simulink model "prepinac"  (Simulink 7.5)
settings: Solver=ode45  StartTime=0.0  StopTime=20  FixedStep=1  MaxStep=1  RelTol=1e-3
libraries: commutil2 x32, dspmtrx3 x28, simulink x20
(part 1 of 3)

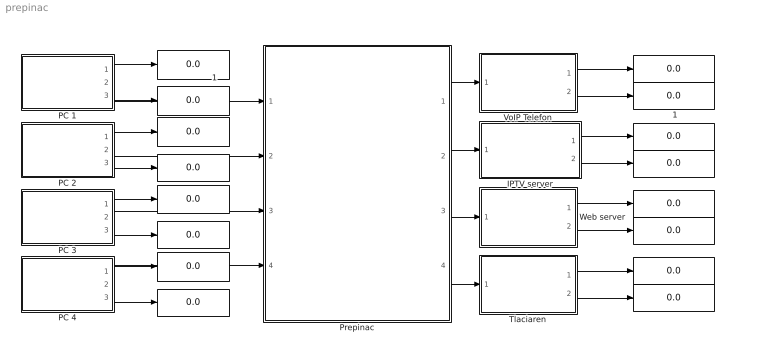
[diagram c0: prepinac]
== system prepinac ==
  " " : Display
  "   " : Display
  "    " : Display
  "     " : Display
  "       " : Display
  "        " : Display
  "          " : Display
  "           " : Display
  "            " : Display
  "                 " : Display
  "                  " : Display
  "                      " : Display
  "                         " : Display
  "                          " : Display
  "                 1" : Display
  " 1" : Display
  IPTV server : Subsystem
  PC 1 : Subsystem
  PC 2 : Subsystem
  PC 3 : Subsystem
  PC 4 : Subsystem
  Prepinac : Subsystem
  Tlaciaren : Subsystem
  VoIP Telefon : Subsystem
  Web server : Subsystem
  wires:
  VoIP Telefon/1(DSCP) -> " "/1
  PC 2/3(MAC) -> "                  "/1
  VoIP Telefon/2(MAC) -> " 1"/1
  IPTV server/2(MAC) -> "     "/1
  Web server/2(MAC) -> "   "/1
  Tlaciaren/2(MAC) -> "        "/1
  IPTV server/1(DSCP) -> "    "/1
  Web server/1(DSCP) -> "          "/1
  Tlaciaren/1(DSCP) -> "            "/1
  PC 1/2(Datovy vystup) -> Prepinac/1(Vstupny port 1)
  PC 4/3(MAC) -> "       "/1
  Prepinac/1(Vystupny port 1) -> VoIP Telefon/1(Vstup)
  Prepinac/3(Vystupny port 3) -> Web server/1(Vstup)
  Prepinac/4(Vystupny port 4) -> Tlaciaren/1(Vstup)
  Prepinac/2(Vystupny port 2) -> IPTV server/1(Vstup)
  PC 3/3(MAC) -> "                         "/1
  PC 1/1(DSCP) -> "                 "/1
  PC 1/3(MAC) -> "                 1"/1
  PC 2/2(Datovy vystup) -> Prepinac/2(Vstupny port 2)
  PC 2/1(DSCP) -> "                      "/1
  PC 3/2(Datovy vystup) -> Prepinac/3(Vstupny port 3)
  PC 3/1(DSCP) -> "                          "/1
  PC 4/1(DSCP) -> "           "/1
  PC 4/2(Datovy vystup) -> Prepinac/4(Vstupny port 4)

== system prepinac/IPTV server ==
  Vstup : Inport  OutDataType=sfix(16)  OutScaling=2^0
  Filtracia DSCP : dspmtrx3/Submatrix  RowSpan=All rows  RowStartMode=Index  RowStartIndex=5  RowEndMode=Index  RowEndIndex=12  ColSpan=Range of columns  ColStartMode=Index  ColStartIndex=113  ColEndMode=Index  ColEndIndex=118
  "MAC adresa " : Constant  Value=[0 0 0 0 0 0 0 0 0 0 1 0 0 1 0 0 1 0 0 1 0 1 1 1 0 0 1 1 0 1 0 0 0 0 0 0 1 1 1 1 1 1 0 0 0 1 0 0]  VectorParams1D=off  OutDataTypeMode=double  OutDataType=sfix(16)  OutScaling=2^0  OutDataTypeStr=double  SampleTime=-1
  Orezanie MAC : dspmtrx3/Submatrix  RowSpan=All rows  RowStartMode=Index  RowStartIndex=5  RowEndMode=Index  RowEndIndex=12  ColSpan=Range of columns  ColStartMode=Index  ColStartIndex=41  ColEndMode=Index  ColEndIndex=48
  Prevod DSCP : commutil2/Bit to Integer Converter  nbits=6  bitOrder=MSB first  signedOutputValues=Unsigned  outDtype=double  outDtypeSigned=Inherit via internal rule
  Prevod MAC : commutil2/Bit to Integer Converter  nbits=8  bitOrder=MSB first  signedOutputValues=Unsigned  outDtype=double  outDtypeSigned=Inherit via internal rule
  DSCP : Outport  OutDataType=sfix(16)  OutScaling=2^0
  MAC : Outport  Port=2  OutDataType=sfix(16)  OutScaling=2^0
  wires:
  Prevod MAC/1 -> MAC/1
  Prevod DSCP/1 -> DSCP/1
  Filtracia DSCP/1 -> Prevod DSCP/1
  Vstup/1 -> Filtracia DSCP/1
  Orezanie MAC/1 -> Prevod MAC/1
  "MAC adresa "/1 -> Orezanie MAC/1

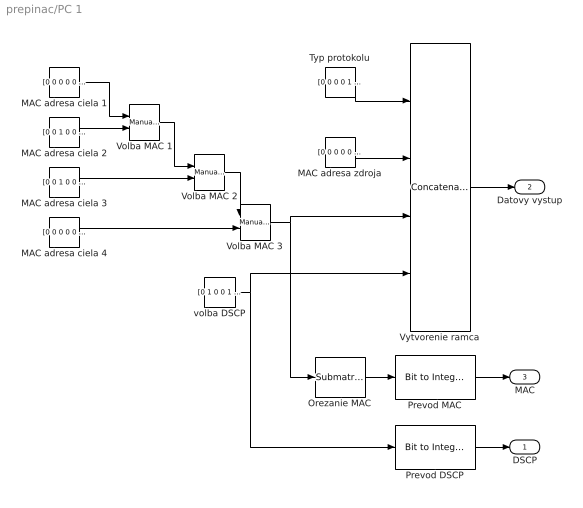
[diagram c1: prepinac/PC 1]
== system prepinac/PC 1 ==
  MAC adresa ciela 1 : Constant  Value=[0 0 0 0 0 0 0 0 0 0 1 0 0 1 0 0 1 0 0 1 0 1 1 1 0 0 1 1 0 1 0 0 0 0 0 0 1 1 1 1 1 1 0 0 0 1 0 0]  VectorParams1D=off  OutDataTypeMode=double  OutDataType=sfix(16)  OutScaling=2^0  OutDataTypeStr=double  SampleTime=-1
  MAC adresa ciela 2 : Constant  Value=[0 0 1 0 0 0 0 0 0 0 0 1 0 1 1 0 1 1 0 1 1 0 0 0 1 1 1 0 0 0 1 1 0 1 1 1 0 0 0 0 1 1 0 0 1 1 1 1]  VectorParams1D=off  OutDataTypeMode=double  OutDataType=sfix(16)  OutScaling=2^0  OutDataTypeStr=double  SampleTime=-1
  MAC adresa ciela 3 : Constant  Value=[0 0 1 0 0 0 0 0 0 0 0 1 0 1 1 0 1 1 0 1 1 0 0 0 1 1 1 0 0 0 1 1 0 1 1 1 0 0 0 0 1 1 0 1 1 1 1 0]  VectorParams1D=off  OutDataTypeMode=double  OutDataType=sfix(16)  OutScaling=2^0  OutDataTypeStr=double  SampleTime=-1
  MAC adresa ciela 4 : Constant  Value=[0 0 0 0 0 0 0 0 0 0 1 1 0 0 0 0 1 1 0 0 0 0 0 1 0 0 1 1 0 0 0 1 0 1 1 1 0 0 1 1 1 0 0 1 1 1 0 1]  VectorParams1D=off  OutDataTypeMode=double  OutDataType=sfix(16)  OutScaling=2^0  OutDataTypeStr=double  SampleTime=-1
  MAC adresa zdroja : Constant  Value=[0 0 0 0 0 0 0 0 0 0 1 0 0 1 0 0 1 0 0 1 0 1 1 1 0 0 1 1 0 1 0 0 0 0 0 0 1 1 1 1 1 1 0 0 0 1 0 1]  VectorParams1D=off  OutDataTypeMode=double  OutDataType=sfix(16)  OutScaling=2^0  OutDataTypeStr=double  SampleTime=-1
  Orezanie MAC : dspmtrx3/Submatrix  RowSpan=All rows  RowStartMode=Index  RowStartIndex=5  RowEndMode=Index  RowEndIndex=12  ColSpan=Range of columns  ColStartMode=Index  ColStartIndex=41  ColEndMode=Index  ColEndIndex=48
  Prevod DSCP : commutil2/Bit to Integer Converter  nbits=6  bitOrder=MSB first  signedOutputValues=Unsigned  outDtype=double  outDtypeSigned=Inherit via internal rule
  Prevod MAC : commutil2/Bit to Integer Converter  nbits=8  bitOrder=MSB first  signedOutputValues=Unsigned  outDtype=double  outDtypeSigned=double
  Typ protokolu : Constant  Value=[0 0 0 0 1 0 0 0 0 0 0 0 0 0 0 0]  VectorParams1D=off  OutDataTypeMode=double  OutDataType=sfix(16)  OutScaling=2^0  OutDataTypeStr=double  SampleTime=-1
  Volba MAC 1 : simulink/Signal Routing/Manual Switch  SystemSampleTime=-1  sw=1  action=0  varsize=off
  Volba MAC 2 : simulink/Signal Routing/Manual Switch  SystemSampleTime=-1  sw=1  action=0  varsize=off
  Volba MAC 3 : simulink/Signal Routing/Manual Switch  SystemSampleTime=-1  sw=1  action=0  varsize=off
  Vytvorenie ramca : Concatenate  NumInputs=4  Mode=Vector
  volba DSCP : Constant  Value=[0 1 0 0 1 0]  VectorParams1D=off  OutDataTypeMode=double  OutDataType=sfix(16)  OutScaling=2^0  OutDataTypeStr=double  SampleTime=-1
  DSCP : Outport  OutDataType=sfix(16)  OutScaling=2^0
  Datovy vystup : Outport  Port=2  OutDataType=sfix(16)  OutScaling=2^0
  MAC : Outport  Port=3  OutDataType=sfix(16)  OutScaling=2^0
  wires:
  Typ protokolu/1 -> Vytvorenie ramca/1
  MAC adresa ciela 2/1 -> Volba MAC 1/2
  MAC adresa ciela 1/1 -> Volba MAC 1/1
  Vytvorenie ramca/1 -> Datovy vystup/1
  MAC adresa ciela 4/1 -> Volba MAC 3/2
  Volba MAC 2/1 -> Volba MAC 3/1
  Volba MAC 1/1 -> Volba MAC 2/1
  MAC adresa ciela 3/1 -> Volba MAC 2/2
  Prevod DSCP/1 -> DSCP/1
  Volba MAC 3/1 -> Vytvorenie ramca/3, Orezanie MAC/1
  Prevod MAC/1 -> MAC/1
  MAC adresa zdroja/1 -> Vytvorenie ramca/2
  volba DSCP/1 -> Vytvorenie ramca/4, Prevod DSCP/1
  Orezanie MAC/1 -> Prevod MAC/1

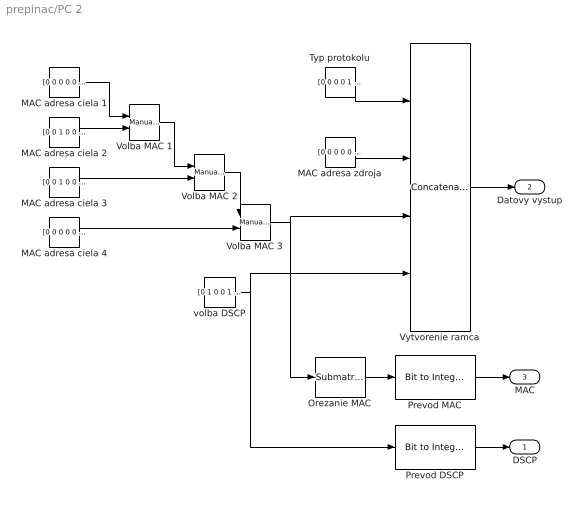
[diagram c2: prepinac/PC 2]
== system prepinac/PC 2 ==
  MAC adresa ciela 1 : Constant  Value=[0 0 0 0 0 0 0 0 0 0 1 0 0 1 0 0 1 0 0 1 0 1 1 1 0 0 1 1 0 1 0 0 0 0 0 0 1 1 1 1 1 1 0 0 0 1 0 0]  VectorParams1D=off  OutDataTypeMode=double  OutDataType=sfix(16)  OutScaling=2^0  OutDataTypeStr=double  SampleTime=-1
  MAC adresa ciela 2 : Constant  Value=[0 0 1 0 0 0 0 0 0 0 0 1 0 1 1 0 1 1 0 1 1 0 0 0 1 1 1 0 0 0 1 1 0 1 1 1 0 0 0 0 1 1 0 0 1 1 1 1]  VectorParams1D=off  OutDataTypeMode=double  OutDataType=sfix(16)  OutScaling=2^0  OutDataTypeStr=double  SampleTime=-1
  MAC adresa ciela 3 : Constant  Value=[0 0 1 0 0 0 0 0 0 0 0 1 0 1 1 0 1 1 0 1 1 0 0 0 1 1 1 0 0 0 1 1 0 1 1 1 0 0 0 0 1 1 0 1 1 1 1 0]  VectorParams1D=off  OutDataTypeMode=double  OutDataType=sfix(16)  OutScaling=2^0  OutDataTypeStr=double  SampleTime=-1
  MAC adresa ciela 4 : Constant  Value=[0 0 0 0 0 0 0 0 0 0 1 1 0 0 0 0 1 1 0 0 0 0 0 1 0 0 1 1 0 0 0 1 0 1 1 1 0 0 1 1 1 0 0 1 1 1 0 1]  VectorParams1D=off  OutDataTypeMode=double  OutDataType=sfix(16)  OutScaling=2^0  OutDataTypeStr=double  SampleTime=-1
  MAC adresa zdroja : Constant  Value=[0 0 0 0 0 0 0 0 0 0 1 0 0 1 0 0 1 0 0 1 0 1 1 1 0 0 1 1 0 1 0 0 0 0 0 0 1 1 1 1 1 1 0 0 0 1 0 1]  VectorParams1D=off  OutDataTypeMode=double  OutDataType=sfix(16)  OutScaling=2^0  OutDataTypeStr=double  SampleTime=-1
  Orezanie MAC : dspmtrx3/Submatrix  RowSpan=All rows  RowStartMode=Index  RowStartIndex=5  RowEndMode=Index  RowEndIndex=12  ColSpan=Range of columns  ColStartMode=Index  ColStartIndex=41  ColEndMode=Index  ColEndIndex=48
  Prevod DSCP : commutil2/Bit to Integer Converter  nbits=6  bitOrder=MSB first  signedOutputValues=Unsigned  outDtype=double  outDtypeSigned=Inherit via internal rule
  Prevod MAC : commutil2/Bit to Integer Converter  nbits=8  bitOrder=MSB first  signedOutputValues=Unsigned  outDtype=double  outDtypeSigned=double
  Typ protokolu : Constant  Value=[0 0 0 0 1 0 0 0 0 0 0 0 0 0 0 0]  VectorParams1D=off  OutDataTypeMode=double  OutDataType=sfix(16)  OutScaling=2^0  OutDataTypeStr=double  SampleTime=-1
  Volba MAC 1 : simulink/Signal Routing/Manual Switch  SystemSampleTime=-1  sw=1  action=0  varsize=off
  Volba MAC 2 : simulink/Signal Routing/Manual Switch  SystemSampleTime=-1  sw=1  action=0  varsize=off
  Volba MAC 3 : simulink/Signal Routing/Manual Switch  SystemSampleTime=-1  sw=1  action=0  varsize=off
  Vytvorenie ramca : Concatenate  NumInputs=4  Mode=Vector
  volba DSCP : Constant  Value=[0 1 0 0 1 0]  VectorParams1D=off  OutDataTypeMode=double  OutDataType=sfix(16)  OutScaling=2^0  OutDataTypeStr=double  SampleTime=-1
  DSCP : Outport  OutDataType=sfix(16)  OutScaling=2^0
  Datovy vystup : Outport  Port=2  OutDataType=sfix(16)  OutScaling=2^0
  MAC : Outport  Port=3  OutDataType=sfix(16)  OutScaling=2^0
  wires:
  Orezanie MAC/1 -> Prevod MAC/1
  volba DSCP/1 -> Prevod DSCP/1, Vytvorenie ramca/4
  MAC adresa zdroja/1 -> Vytvorenie ramca/2
  Prevod MAC/1 -> MAC/1
  Volba MAC 3/1 -> Orezanie MAC/1, Vytvorenie ramca/3
  Prevod DSCP/1 -> DSCP/1
  MAC adresa ciela 3/1 -> Volba MAC 2/2
  Volba MAC 1/1 -> Volba MAC 2/1
  Volba MAC 2/1 -> Volba MAC 3/1
  MAC adresa ciela 4/1 -> Volba MAC 3/2
  Vytvorenie ramca/1 -> Datovy vystup/1
  MAC adresa ciela 1/1 -> Volba MAC 1/1
  MAC adresa ciela 2/1 -> Volba MAC 1/2
  Typ protokolu/1 -> Vytvorenie ramca/1

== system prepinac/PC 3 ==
  MAC adresa ciela 1 : Constant  Value=[0 0 0 0 0 0 0 0 0 0 1 0 0 1 0 0 1 0 0 1 0 1 1 1 0 0 1 1 0 1 0 0 0 0 0 0 1 1 1 1 1 1 0 0 0 1 0 0]  VectorParams1D=off  OutDataTypeMode=double  OutDataType=sfix(16)  OutScaling=2^0  OutDataTypeStr=double  SampleTime=-1
  MAC adresa ciela 2 : Constant  Value=[0 0 1 0 0 0 0 0 0 0 0 1 0 1 1 0 1 1 0 1 1 0 0 0 1 1 1 0 0 0 1 1 0 1 1 1 0 0 0 0 1 1 0 0 1 1 1 1]  VectorParams1D=off  OutDataTypeMode=double  OutDataType=sfix(16)  OutScaling=2^0  OutDataTypeStr=double  SampleTime=-1
  MAC adresa ciela 3 : Constant  Value=[0 0 1 0 0 0 0 0 0 0 0 1 0 1 1 0 1 1 0 1 1 0 0 0 1 1 1 0 0 0 1 1 0 1 1 1 0 0 0 0 1 1 0 1 1 1 1 0]  VectorParams1D=off  OutDataTypeMode=double  OutDataType=sfix(16)  OutScaling=2^0  OutDataTypeStr=double  SampleTime=-1
  MAC adresa ciela 4 : Constant  Value=[0 0 0 0 0 0 0 0 0 0 1 1 0 0 0 0 1 1 0 0 0 0 0 1 0 0 1 1 0 0 0 1 0 1 1 1 0 0 1 1 1 0 0 1 1 1 0 1]  VectorParams1D=off  OutDataTypeMode=double  OutDataType=sfix(16)  OutScaling=2^0  OutDataTypeStr=double  SampleTime=-1
  MAC adresa zdroja : Constant  Value=[0 0 0 0 0 0 0 0 0 0 1 0 0 1 0 0 1 0 0 1 0 1 1 1 0 0 1 1 0 1 0 0 0 0 0 0 1 1 1 1 1 1 0 0 0 1 0 1]  VectorParams1D=off  OutDataTypeMode=double  OutDataType=sfix(16)  OutScaling=2^0  OutDataTypeStr=double  SampleTime=-1
  Orezanie MAC : dspmtrx3/Submatrix  RowSpan=All rows  RowStartMode=Index  RowStartIndex=5  RowEndMode=Index  RowEndIndex=12  ColSpan=Range of columns  ColStartMode=Index  ColStartIndex=41  ColEndMode=Index  ColEndIndex=48
  Prevod DSCP : commutil2/Bit to Integer Converter  nbits=6  bitOrder=MSB first  signedOutputValues=Unsigned  outDtype=double  outDtypeSigned=Inherit via internal rule
  Prevod MAC : commutil2/Bit to Integer Converter  nbits=8  bitOrder=MSB first  signedOutputValues=Unsigned  outDtype=double  outDtypeSigned=double
  Typ protokolu : Constant  Value=[0 0 0 0 1 0 0 0 0 0 0 0 0 0 0 0]  VectorParams1D=off  OutDataTypeMode=double  OutDataType=sfix(16)  OutScaling=2^0  OutDataTypeStr=double  SampleTime=-1
  Volba MAC 1 : simulink/Signal Routing/Manual Switch  SystemSampleTime=-1  sw=1  action=0  varsize=off
  Volba MAC 2 : simulink/Signal Routing/Manual Switch  SystemSampleTime=-1  sw=1  action=0  varsize=off
  Volba MAC 3 : simulink/Signal Routing/Manual Switch  SystemSampleTime=-1  sw=1  action=0  varsize=off
  Vytvorenie ramca : Concatenate  NumInputs=4  Mode=Vector
  volba DSCP : Constant  Value=[0 1 0 0 1 0]  VectorParams1D=off  OutDataTypeMode=double  OutDataType=sfix(16)  OutScaling=2^0  OutDataTypeStr=double  SampleTime=-1
  DSCP : Outport  OutDataType=sfix(16)  OutScaling=2^0
  Datovy vystup : Outport  Port=2  OutDataType=sfix(16)  OutScaling=2^0
  MAC : Outport  Port=3  OutDataType=sfix(16)  OutScaling=2^0
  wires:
  Typ protokolu/1 -> Vytvorenie ramca/1
  MAC adresa ciela 2/1 -> Volba MAC 1/2
  MAC adresa ciela 1/1 -> Volba MAC 1/1
  Vytvorenie ramca/1 -> Datovy vystup/1
  MAC adresa ciela 4/1 -> Volba MAC 3/2
  Volba MAC 2/1 -> Volba MAC 3/1
  Volba MAC 1/1 -> Volba MAC 2/1
  MAC adresa ciela 3/1 -> Volba MAC 2/2
  Prevod DSCP/1 -> DSCP/1
  Volba MAC 3/1 -> Vytvorenie ramca/3, Orezanie MAC/1
  Prevod MAC/1 -> MAC/1
  MAC adresa zdroja/1 -> Vytvorenie ramca/2
  volba DSCP/1 -> Vytvorenie ramca/4, Prevod DSCP/1
  Orezanie MAC/1 -> Prevod MAC/1

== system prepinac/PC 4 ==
  MAC adresa ciela 1 : Constant  Value=[0 0 0 0 0 0 0 0 0 0 1 0 0 1 0 0 1 0 0 1 0 1 1 1 0 0 1 1 0 1 0 0 0 0 0 0 1 1 1 1 1 1 0 0 0 1 0 0]  VectorParams1D=off  OutDataTypeMode=double  OutDataType=sfix(16)  OutScaling=2^0  OutDataTypeStr=double  SampleTime=-1
  MAC adresa ciela 2 : Constant  Value=[0 0 1 0 0 0 0 0 0 0 0 1 0 1 1 0 1 1 0 1 1 0 0 0 1 1 1 0 0 0 1 1 0 1 1 1 0 0 0 0 1 1 0 0 1 1 1 1]  VectorParams1D=off  OutDataTypeMode=double  OutDataType=sfix(16)  OutScaling=2^0  OutDataTypeStr=double  SampleTime=-1
  MAC adresa ciela 3 : Constant  Value=[0 0 1 0 0 0 0 0 0 0 0 1 0 1 1 0 1 1 0 1 1 0 0 0 1 1 1 0 0 0 1 1 0 1 1 1 0 0 0 0 1 1 0 1 1 1 1 0]  VectorParams1D=off  OutDataTypeMode=double  OutDataType=sfix(16)  OutScaling=2^0  OutDataTypeStr=double  SampleTime=-1
  MAC adresa ciela 4 : Constant  Value=[0 0 0 0 0 0 0 0 0 0 1 1 0 0 0 0 1 1 0 0 0 0 0 1 0 0 1 1 0 0 0 1 0 1 1 1 0 0 1 1 1 0 0 1 1 1 0 1]  VectorParams1D=off  OutDataTypeMode=double  OutDataType=sfix(16)  OutScaling=2^0  OutDataTypeStr=double  SampleTime=-1
  MAC adresa zdroja : Constant  Value=[0 0 0 0 0 0 0 0 0 0 1 0 0 1 0 0 1 0 0 1 0 1 1 1 0 0 1 1 0 1 0 0 0 0 0 0 1 1 1 1 1 1 0 0 0 1 0 1]  VectorParams1D=off  OutDataTypeMode=double  OutDataType=sfix(16)  OutScaling=2^0  OutDataTypeStr=double  SampleTime=-1
  Orezanie MAC : dspmtrx3/Submatrix  RowSpan=All rows  RowStartMode=Index  RowStartIndex=5  RowEndMode=Index  RowEndIndex=12  ColSpan=Range of columns  ColStartMode=Index  ColStartIndex=41  ColEndMode=Index  ColEndIndex=48
  Prevod DSCP : commutil2/Bit to Integer Converter  nbits=6  bitOrder=MSB first  signedOutputValues=Unsigned  outDtype=double  outDtypeSigned=Inherit via internal rule
  Prevod MAC : commutil2/Bit to Integer Converter  nbits=8  bitOrder=MSB first  signedOutputValues=Unsigned  outDtype=double  outDtypeSigned=double
  Typ protokolu : Constant  Value=[0 0 0 0 1 0 0 0 0 0 0 0 0 0 0 0]  VectorParams1D=off  OutDataTypeMode=double  OutDataType=sfix(16)  OutScaling=2^0  OutDataTypeStr=double  SampleTime=-1
  Volba MAC 1 : simulink/Signal Routing/Manual Switch  SystemSampleTime=-1  sw=1  action=0  varsize=off
  Volba MAC 2 : simulink/Signal Routing/Manual Switch  SystemSampleTime=-1  sw=1  action=0  varsize=off
  Volba MAC 3 : simulink/Signal Routing/Manual Switch  SystemSampleTime=-1  sw=1  action=0  varsize=off
  Vytvorenie ramca : Concatenate  NumInputs=4  Mode=Vector
  volba DSCP : Constant  Value=[0 1 0 0 1 0]  VectorParams1D=off  OutDataTypeMode=double  OutDataType=sfix(16)  OutScaling=2^0  OutDataTypeStr=double  SampleTime=-1
  DSCP : Outport  OutDataType=sfix(16)  OutScaling=2^0
  Datovy vystup : Outport  Port=2  OutDataType=sfix(16)  OutScaling=2^0
  MAC : Outport  Port=3  OutDataType=sfix(16)  OutScaling=2^0
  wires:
  Orezanie MAC/1 -> Prevod MAC/1
  volba DSCP/1 -> Prevod DSCP/1, Vytvorenie ramca/4
  MAC adresa zdroja/1 -> Vytvorenie ramca/2
  Prevod MAC/1 -> MAC/1
  Volba MAC 3/1 -> Orezanie MAC/1, Vytvorenie ramca/3
  Prevod DSCP/1 -> DSCP/1
  MAC adresa ciela 3/1 -> Volba MAC 2/2
  Volba MAC 1/1 -> Volba MAC 2/1
  Volba MAC 2/1 -> Volba MAC 3/1
  MAC adresa ciela 4/1 -> Volba MAC 3/2
  Vytvorenie ramca/1 -> Datovy vystup/1
  MAC adresa ciela 1/1 -> Volba MAC 1/1
  MAC adresa ciela 2/1 -> Volba MAC 1/2
  Typ protokolu/1 -> Vytvorenie ramca/1

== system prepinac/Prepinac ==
  Vstupny port 1 : Inport  OutDataType=sfix(16)  OutScaling=2^0
  Vstupny port 2 : Inport  Port=2  OutDataType=sfix(16)  OutScaling=2^0
  Vstupny port 3 : Inport  Port=3  OutDataType=sfix(16)  OutScaling=2^0
  Vstupny port 4 : Inport  Port=4  OutDataType=sfix(16)  OutScaling=2^0
  Riadenie QoS : Subsystem
  Riadenie prepinania : Subsystem
  Vystupny port 1 : Outport  OutDataType=sfix(16)  OutScaling=2^0
  Vystupny port 2 : Outport  Port=2  OutDataType=sfix(16)  OutScaling=2^0
  Vystupny port 3 : Outport  Port=3  OutDataType=sfix(16)  OutScaling=2^0
  Vystupny port 4 : Outport  Port=4  OutDataType=sfix(16)  OutScaling=2^0
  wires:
  Vstupny port 1/1 -> Riadenie QoS/1(In1), Riadenie prepinania/1(MAC1)
  Vstupny port 2/1 -> Riadenie QoS/2(In2), Riadenie prepinania/2(MAC2)
  Vstupny port 3/1 -> Riadenie QoS/3(In3), Riadenie prepinania/3(MAC3)
  Vstupny port 4/1 -> Riadenie QoS/4(In4), Riadenie prepinania/4(MAC4)
  Riadenie QoS/1(Datovy vystup) -> Riadenie prepinania/5(Data)
  Riadenie prepinania/4(Vystup4) -> Vystupny port 4/1
  Riadenie prepinania/3(Vystup3) -> Vystupny port 3/1
  Riadenie prepinania/2(Vystup2) -> Vystupny port 2/1
  Riadenie prepinania/1(Vystup1) -> Vystupny port 1/1

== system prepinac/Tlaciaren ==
  Vstup : Inport  OutDataType=sfix(16)  OutScaling=2^0
  Filtracia DSCP : dspmtrx3/Submatrix  RowSpan=All rows  RowStartMode=Index  RowStartIndex=5  RowEndMode=Index  RowEndIndex=12  ColSpan=Range of columns  ColStartMode=Index  ColStartIndex=113  ColEndMode=Index  ColEndIndex=118
  "MAC adresa " : Constant  Value=[0 0 0 0 0 0 0 0 0 0 1 0 0 1 0 0 1 0 0 1 0 1 1 1 0 0 1 1 0 1 0 0 0 0 0 0 1 1 1 1 1 1 0 0 0 1 0 0]  VectorParams1D=off  OutDataTypeMode=double  OutDataType=sfix(16)  OutScaling=2^0  OutDataTypeStr=double  SampleTime=-1
  Orezanie MAC : dspmtrx3/Submatrix  RowSpan=All rows  RowStartMode=Index  RowStartIndex=5  RowEndMode=Index  RowEndIndex=12  ColSpan=Range of columns  ColStartMode=Index  ColStartIndex=41  ColEndMode=Index  ColEndIndex=48
  Prevod DSCP : commutil2/Bit to Integer Converter  nbits=6  bitOrder=MSB first  signedOutputValues=Unsigned  outDtype=double  outDtypeSigned=Inherit via internal rule
  Prevod MAC : commutil2/Bit to Integer Converter  nbits=8  bitOrder=MSB first  signedOutputValues=Unsigned  outDtype=double  outDtypeSigned=Inherit via internal rule
  DSCP : Outport  OutDataType=sfix(16)  OutScaling=2^0
  MAC : Outport  Port=2  OutDataType=sfix(16)  OutScaling=2^0
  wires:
  Prevod MAC/1 -> MAC/1
  Prevod DSCP/1 -> DSCP/1
  Filtracia DSCP/1 -> Prevod DSCP/1
  Vstup/1 -> Filtracia DSCP/1
  Orezanie MAC/1 -> Prevod MAC/1
  "MAC adresa "/1 -> Orezanie MAC/1

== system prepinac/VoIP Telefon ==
  Vstup : Inport  OutDataType=sfix(16)  OutScaling=2^0
  Filtracia DSCP : dspmtrx3/Submatrix  RowSpan=All rows  RowStartMode=Index  RowStartIndex=5  RowEndMode=Index  RowEndIndex=12  ColSpan=Range of columns  ColStartMode=Index  ColStartIndex=113  ColEndMode=Index  ColEndIndex=118
  "MAC adresa " : Constant  Value=[0 0 0 0 0 0 0 0 0 0 1 0 0 1 0 0 1 0 0 1 0 1 1 1 0 0 1 1 0 1 0 0 0 0 0 0 1 1 1 1 1 1 0 0 0 1 0 0]  VectorParams1D=off  OutDataTypeMode=double  OutDataType=sfix(16)  OutScaling=2^0  OutDataTypeStr=double  SampleTime=-1
  Orezanie MAC : dspmtrx3/Submatrix  RowSpan=All rows  RowStartMode=Index  RowStartIndex=5  RowEndMode=Index  RowEndIndex=12  ColSpan=Range of columns  ColStartMode=Index  ColStartIndex=41  ColEndMode=Index  ColEndIndex=48
  Prevod DSCP : commutil2/Bit to Integer Converter  nbits=6  bitOrder=MSB first  signedOutputValues=Unsigned  outDtype=double  outDtypeSigned=Inherit via internal rule
  Prevod MAC : commutil2/Bit to Integer Converter  nbits=8  bitOrder=MSB first  signedOutputValues=Unsigned  outDtype=double  outDtypeSigned=Inherit via internal rule
  DSCP : Outport  OutDataType=sfix(16)  OutScaling=2^0
  MAC : Outport  Port=2  OutDataType=sfix(16)  OutScaling=2^0
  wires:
  "MAC adresa "/1 -> Orezanie MAC/1
  Orezanie MAC/1 -> Prevod MAC/1
  Vstup/1 -> Filtracia DSCP/1
  Filtracia DSCP/1 -> Prevod DSCP/1
  Prevod DSCP/1 -> DSCP/1
  Prevod MAC/1 -> MAC/1

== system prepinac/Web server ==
  Vstup : Inport  OutDataType=sfix(16)  OutScaling=2^0
  Filtracia DSCP : dspmtrx3/Submatrix  RowSpan=All rows  RowStartMode=Index  RowStartIndex=5  RowEndMode=Index  RowEndIndex=12  ColSpan=Range of columns  ColStartMode=Index  ColStartIndex=113  ColEndMode=Index  ColEndIndex=118
  "MAC adresa " : Constant  Value=[0 0 0 0 0 0 0 0 0 0 1 0 0 1 0 0 1 0 0 1 0 1 1 1 0 0 1 1 0 1 0 0 0 0 0 0 1 1 1 1 1 1 0 0 0 1 0 0]  VectorParams1D=off  OutDataTypeMode=double  OutDataType=sfix(16)  OutScaling=2^0  OutDataTypeStr=double  SampleTime=-1
  Orezanie MAC : dspmtrx3/Submatrix  RowSpan=All rows  RowStartMode=Index  RowStartIndex=5  RowEndMode=Index  RowEndIndex=12  ColSpan=Range of columns  ColStartMode=Index  ColStartIndex=41  ColEndMode=Index  ColEndIndex=48
  Prevod DSCP : commutil2/Bit to Integer Converter  nbits=6  bitOrder=MSB first  signedOutputValues=Unsigned  outDtype=double  outDtypeSigned=Inherit via internal rule
  Prevod MAC : commutil2/Bit to Integer Converter  nbits=8  bitOrder=MSB first  signedOutputValues=Unsigned  outDtype=double  outDtypeSigned=Inherit via internal rule
  DSCP : Outport  OutDataType=sfix(16)  OutScaling=2^0
  MAC : Outport  Port=2  OutDataType=sfix(16)  OutScaling=2^0
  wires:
  "MAC adresa "/1 -> Orezanie MAC/1
  Orezanie MAC/1 -> Prevod MAC/1
  Vstup/1 -> Filtracia DSCP/1
  Filtracia DSCP/1 -> Prevod DSCP/1
  Prevod DSCP/1 -> DSCP/1
  Prevod MAC/1 -> MAC/1

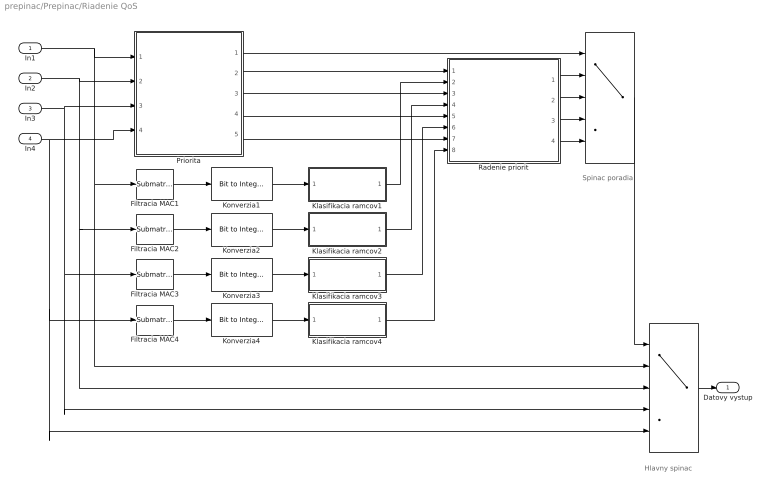
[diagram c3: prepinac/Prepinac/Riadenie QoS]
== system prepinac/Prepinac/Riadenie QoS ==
  note: Hlavny spinac
  note: Spinac poradia
  In1 : Inport  OutDataType=sfix(16)  OutScaling=2^0
  In2 : Inport  Port=2  OutDataType=sfix(16)  OutScaling=2^0
  In3 : Inport  Port=3  OutDataType=sfix(16)  OutScaling=2^0
  In4 : Inport  Port=4  OutDataType=sfix(16)  OutScaling=2^0
  "   " : MultiPortSwitch  DataPortOrder=Zero-based contiguous  Inputs=4  zeroidx=on
  "         " : MultiPortSwitch  Inputs=4  zeroidx=off
  Filtracia MAC{1..4} (4 alike) : dspmtrx3/Submatrix  RowSpan=All rows  RowStartMode=Index  RowStartIndex=5  RowEndMode=Index  RowEndIndex=12  ColSpan=Range of columns  ColStartMode=Index  ColStartIndex=105  ColEndMode=Index  ColEndIndex=112
  Klasifikacia ramcov1 : Subsystem
  Klasifikacia ramcov2 : Subsystem
  Klasifikacia ramcov3 : Subsystem
  Klasifikacia ramcov4 : Subsystem
  Konverzia{1..4} (4 alike) : commutil2/Bit to Integer Converter  nbits=8  bitOrder=MSB first  signedOutputValues=Unsigned  outDtype=Same as input  outDtypeSigned=Inherit via internal rule
  Priorita : Subsystem
  Radenie priorit : Subsystem
  Datovy vystup : Outport  OutDataType=sfix(16)  OutScaling=2^0
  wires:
  In1/1 -> Priorita/1(In1), "         "/2, Filtracia MAC1/1
  In2/1 -> Priorita/2(In2), "         "/3, Filtracia MAC2/1
  In3/1 -> Priorita/3(In3), "         "/4, Filtracia MAC3/1
  In4/1 -> Priorita/4(In4), "         "/5, Filtracia MAC4/1
  "         "/1 -> Datovy vystup/1
  Priorita/2(Out1) -> Radenie priorit/1(vst1)
  Priorita/3(Out2) -> Radenie priorit/3(vst2)
  Priorita/4(Out3) -> Radenie priorit/5(vst3)
  Priorita/5(Out4) -> Radenie priorit/7(vst4)
  Priorita/1(Trg1) -> "   "/1
  Radenie priorit/1(sig1) -> "   "/2
  Radenie priorit/2(sig2) -> "   "/3
  Radenie priorit/3(sig3) -> "   "/4
  Radenie priorit/4(sig4) -> "   "/5
  "   "/1 -> "         "/1
  Filtracia MAC1/1 -> Konverzia1/1
  Filtracia MAC2/1 -> Konverzia2/1
  Filtracia MAC3/1 -> Konverzia3/1
  Filtracia MAC4/1 -> Konverzia4/1
  Konverzia1/1 -> Klasifikacia ramcov1/1(In)
  Konverzia2/1 -> Klasifikacia ramcov2/1(In)
  Konverzia3/1 -> Klasifikacia ramcov3/1(In)
  Konverzia4/1 -> Klasifikacia ramcov4/1(In)
  Klasifikacia ramcov4/1(Out) -> Radenie priorit/8(adr4)
  Klasifikacia ramcov3/1(Out) -> Radenie priorit/6(adr3)
  Klasifikacia ramcov2/1(Out) -> Radenie priorit/4(adr2)
  Klasifikacia ramcov1/1(Out) -> Radenie priorit/2(adr1)

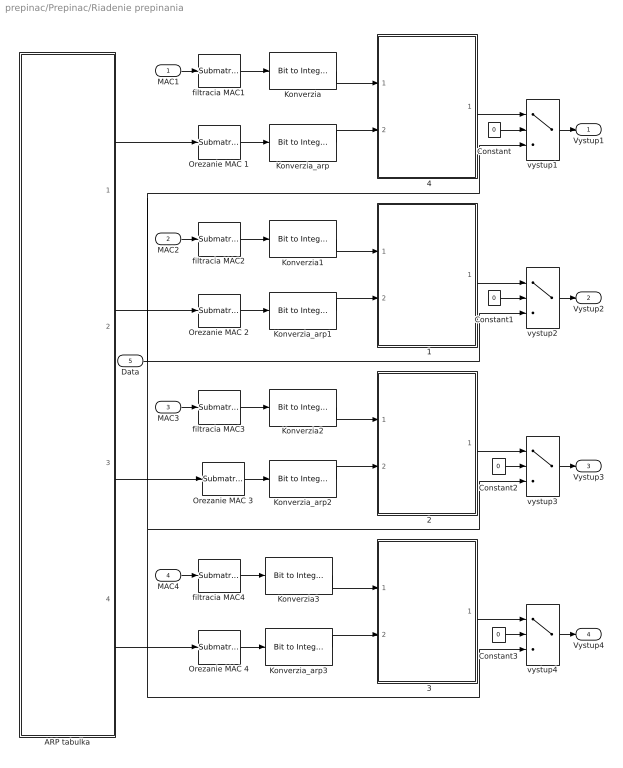
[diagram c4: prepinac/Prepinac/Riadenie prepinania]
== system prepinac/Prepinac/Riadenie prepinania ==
  MAC1 : Inport  OutDataType=sfix(16)  OutScaling=2^0
  MAC2 : Inport  Port=2  OutDataType=sfix(16)  OutScaling=2^0
  MAC3 : Inport  Port=3  OutDataType=sfix(16)  OutScaling=2^0
  MAC4 : Inport  Port=4  OutDataType=sfix(16)  OutScaling=2^0
  Data : Inport  Port=5  OutDataType=sfix(16)  OutScaling=2^0
  "  1" : Stateflow chart  TreatAsAtomicUnit=on
  "  2" : Stateflow chart  TreatAsAtomicUnit=on
  "  3" : Stateflow chart  TreatAsAtomicUnit=on
  "  4" : Stateflow chart  TreatAsAtomicUnit=on
  ARP tabulka : Subsystem
  Constant{,1..3} (4 alike) : Constant  Value=0  OutDataType=sfix(16)  OutScaling=2^0
  Konverzia{,1..3} (4 alike) : commutil2/Bit to Integer Converter  nbits=8  bitOrder=MSB first  signedOutputValues=Unsigned  outDtype=Same as input  outDtypeSigned=Inherit via internal rule
  Konverzia_arp{,1..3} (4 alike) : commutil2/Bit to Integer Converter  nbits=8  bitOrder=MSB first  signedOutputValues=Unsigned  outDtype=double  outDtypeSigned=Inherit via internal rule
  Orezanie MAC {1..4} (4 alike) : dspmtrx3/Submatrix  RowSpan=All rows  RowStartMode=Index  RowStartIndex=5  RowEndMode=Index  RowEndIndex=12  ColSpan=Range of columns  ColStartMode=Index  ColStartIndex=41  ColEndMode=Index  ColEndIndex=48
  filtracia MAC{1..4} (4 alike) : dspmtrx3/Submatrix  RowSpan=All rows  RowStartMode=Index  RowStartIndex=5  RowEndMode=Index  RowEndIndex=12  ColSpan=Range of columns  ColStartMode=Index  ColStartIndex=105  ColEndMode=Index  ColEndIndex=112
  vystup{1..4} (4 alike) : MultiPortSwitch  Inputs=2  zeroidx=off
  Vystup1 : Outport  OutDataType=sfix(16)  OutScaling=2^0
  Vystup2 : Outport  Port=2  OutDataType=sfix(16)  OutScaling=2^0
  Vystup3 : Outport  Port=3  OutDataType=sfix(16)  OutScaling=2^0
  Vystup4 : Outport  Port=4  OutDataType=sfix(16)  OutScaling=2^0
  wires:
  vystup2/1 -> Vystup2/1
  vystup1/1 -> Vystup1/1
  Data/1 -> vystup1/3, vystup3/3, vystup4/3, vystup2/3
  vystup3/1 -> Vystup3/1
  vystup4/1 -> Vystup4/1
  Constant/1 -> vystup1/2
  Constant1/1 -> vystup2/2
  Orezanie MAC 1/1 -> Konverzia_arp/1
  Orezanie MAC 2/1 -> Konverzia_arp1/1
  Orezanie MAC 3/1 -> Konverzia_arp2/1
  Orezanie MAC 4/1 -> Konverzia_arp3/1
  ARP tabulka/1(MAC adresa 1) -> Orezanie MAC 1/1
  ARP tabulka/4(MAC adresa 4) -> Orezanie MAC 4/1
  ARP tabulka/3(MAC adresa 3) -> Orezanie MAC 3/1
  ARP tabulka/2(MAC adresa 2) -> Orezanie MAC 2/1
  filtracia MAC1/1 -> Konverzia/1
  filtracia MAC2/1 -> Konverzia1/1
  filtracia MAC3/1 -> Konverzia2/1
  filtracia MAC4/1 -> Konverzia3/1
  Konverzia1/1 -> "  1"/1(MAC_prijata)
  Konverzia2/1 -> "  2"/1(MAC_prijata)
  Konverzia3/1 -> "  3"/1(MAC_prijata)
  MAC1/1 -> filtracia MAC1/1
  MAC2/1 -> filtracia MAC2/1
  MAC3/1 -> filtracia MAC3/1
  MAC4/1 -> filtracia MAC4/1
  Konverzia_arp2/1 -> "  2"/2(MAC_arp)
  Konverzia_arp1/1 -> "  1"/2(MAC_arp)
  Konverzia_arp/1 -> "  4"/2(MAC_arp)
  Konverzia/1 -> "  4"/1(MAC_prijata)
  "  4"/1(y) -> vystup1/1
  Konverzia_arp3/1 -> "  3"/2(MAC_arp)
  "  1"/1(y) -> vystup2/1
  "  2"/1(y) -> vystup3/1
  Constant2/1 -> vystup3/2
  "  3"/1(y) -> vystup4/1
  Constant3/1 -> vystup4/2

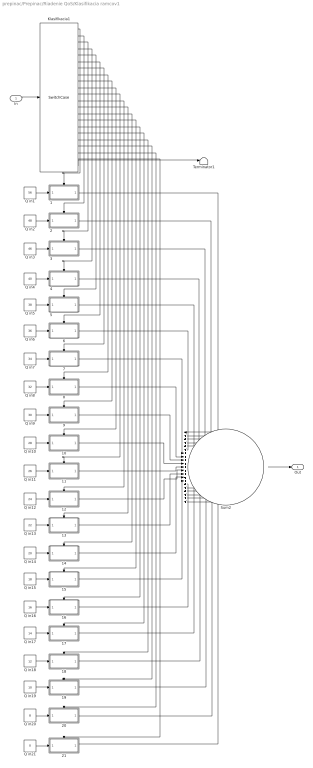
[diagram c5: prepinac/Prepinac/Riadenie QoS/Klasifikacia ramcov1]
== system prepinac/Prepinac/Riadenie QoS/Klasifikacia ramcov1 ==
  In : Inport  OutDataType=sfix(16)  OutScaling=2^0
  1 : Subsystem  TreatAsAtomicUnit=on
  10 : Subsystem  TreatAsAtomicUnit=on
  11 : Subsystem  TreatAsAtomicUnit=on
  12 : Subsystem  TreatAsAtomicUnit=on
  13 : Subsystem  TreatAsAtomicUnit=on
  14 : Subsystem  TreatAsAtomicUnit=on
  15 : Subsystem  TreatAsAtomicUnit=on
  16 : Subsystem  TreatAsAtomicUnit=on
  17 : Subsystem  TreatAsAtomicUnit=on
  18 : Subsystem  TreatAsAtomicUnit=on
  19 : Subsystem  TreatAsAtomicUnit=on
  2 : Subsystem  TreatAsAtomicUnit=on
  20 : Subsystem  TreatAsAtomicUnit=on
  21 : Subsystem  TreatAsAtomicUnit=on
  3 : Subsystem  TreatAsAtomicUnit=on
  4 : Subsystem  TreatAsAtomicUnit=on
  5 : Subsystem  TreatAsAtomicUnit=on
  6 : Subsystem  TreatAsAtomicUnit=on
  7 : Subsystem  TreatAsAtomicUnit=on
  8 : Subsystem  TreatAsAtomicUnit=on
  9 : Subsystem  TreatAsAtomicUnit=on
  Klasifikacia1 : SwitchCase  CaseConditions={0,8,10,12,14,16,18,20,22,24,26,28,30,32,34,36,38,40,46,48,56}
  Q in1 : Constant  Value=56  VectorParams1D=off  OutDataTypeMode=double  OutDataType=sfix(16)  OutScaling=2^0  OutDataTypeStr=double  SampleTime=-1
  Q in10 : Constant  Value=28  VectorParams1D=off  OutDataTypeMode=double  OutDataType=sfix(16)  OutScaling=2^0  OutDataTypeStr=double  SampleTime=-1
  Q in11 : Constant  Value=26  VectorParams1D=off  OutDataTypeMode=double  OutDataType=sfix(16)  OutScaling=2^0  OutDataTypeStr=double  SampleTime=-1
  Q in12 : Constant  Value=24  VectorParams1D=off  OutDataTypeMode=double  OutDataType=sfix(16)  OutScaling=2^0  OutDataTypeStr=double  SampleTime=-1
  Q in13 : Constant  Value=22  VectorParams1D=off  OutDataTypeMode=double  OutDataType=sfix(16)  OutScaling=2^0  OutDataTypeStr=double  SampleTime=-1
  Q in14 : Constant  Value=20  VectorParams1D=off  OutDataTypeMode=double  OutDataType=sfix(16)  OutScaling=2^0  OutDataTypeStr=double  SampleTime=-1
  Q in15 : Constant  Value=18  VectorParams1D=off  OutDataTypeMode=double  OutDataType=sfix(16)  OutScaling=2^0  OutDataTypeStr=double  SampleTime=-1
  Q in16 : Constant  Value=16  VectorParams1D=off  OutDataTypeMode=double  OutDataType=sfix(16)  OutScaling=2^0  OutDataTypeStr=double  SampleTime=-1
  Q in17 : Constant  Value=14  VectorParams1D=off  OutDataTypeMode=double  OutDataType=sfix(16)  OutScaling=2^0  OutDataTypeStr=double  SampleTime=-1
  Q in18 : Constant  Value=12  VectorParams1D=off  OutDataTypeMode=double  OutDataType=sfix(16)  OutScaling=2^0  OutDataTypeStr=double  SampleTime=-1
  Q in19 : Constant  Value=10  VectorParams1D=off  OutDataTypeMode=double  OutDataType=sfix(16)  OutScaling=2^0  OutDataTypeStr=double  SampleTime=-1
  Q in2 : Constant  Value=48  VectorParams1D=off  OutDataTypeMode=double  OutDataType=sfix(16)  OutScaling=2^0  OutDataTypeStr=double  SampleTime=-1
  Q in20 : Constant  Value=8  VectorParams1D=off  OutDataTypeMode=double  OutDataType=sfix(16)  OutScaling=2^0  OutDataTypeStr=double  SampleTime=-1
  Q in21 : Constant  Value=0  VectorParams1D=off  OutDataTypeMode=double  OutDataType=sfix(16)  OutScaling=2^0  OutDataTypeStr=double  SampleTime=-1
  Q in3 : Constant  Value=46  VectorParams1D=off  OutDataTypeMode=double  OutDataType=sfix(16)  OutScaling=2^0  OutDataTypeStr=double  SampleTime=-1
  Q in4 : Constant  Value=40  VectorParams1D=off  OutDataTypeMode=double  OutDataType=sfix(16)  OutScaling=2^0  OutDataTypeStr=double  SampleTime=-1
  Q in5 : Constant  Value=38  VectorParams1D=off  OutDataTypeMode=double  OutDataType=sfix(16)  OutScaling=2^0  OutDataTypeStr=double  SampleTime=-1
  Q in6 : Constant  Value=36  VectorParams1D=off  OutDataTypeMode=double  OutDataType=sfix(16)  OutScaling=2^0  OutDataTypeStr=double  SampleTime=-1
  Q in7 : Constant  Value=34  VectorParams1D=off  OutDataTypeMode=double  OutDataType=sfix(16)  OutScaling=2^0  OutDataTypeStr=double  SampleTime=-1
  Q in8 : Constant  Value=32  VectorParams1D=off  OutDataTypeMode=double  OutDataType=sfix(16)  OutScaling=2^0  OutDataTypeStr=double  SampleTime=-1
  Q in9 : Constant  Value=30  VectorParams1D=off  OutDataTypeMode=double  OutDataType=sfix(16)  OutScaling=2^0  OutDataTypeStr=double  SampleTime=-1
  Sum2 : Sum  Inputs=|+++++++++++++++++++++  OutDataType=sfix(16)  OutScaling=2^0
  Terminator1 : Terminator
  Out : Outport  OutDataType=sfix(16)  OutScaling=2^0
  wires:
  1/1(Out1) -> Sum2/1
  2/1(Out1) -> Sum2/2
  3/1(Out1) -> Sum2/3
  4/1(Out1) -> Sum2/4
  Q in1/1 -> 1/1(In1)
  Q in2/1 -> 2/1(In1)
  Q in3/1 -> 3/1(In1)
  Q in4/1 -> 4/1(In1)
  Q in5/1 -> 5/1(In1)
  Q in6/1 -> 6/1(In1)
  Q in7/1 -> 7/1(In1)
  Q in8/1 -> 8/1(In1)
  Q in9/1 -> 9/1(In1)
  Q in10/1 -> 10/1(In1)
  Q in11/1 -> 11/1(In1)
  Q in12/1 -> 12/1(In1)
  Q in13/1 -> 13/1(In1)
  Q in14/1 -> 14/1(In1)
  Q in15/1 -> 15/1(In1)
  Q in16/1 -> 16/1(In1)
  Q in17/1 -> 17/1(In1)
  Q in18/1 -> 18/1(In1)
  Q in19/1 -> 19/1(In1)
  Q in20/1 -> 20/1(In1)
  Q in21/1 -> 21/1(In1)
  5/1(Out1) -> Sum2/5
  6/1(Out1) -> Sum2/6
  7/1(Out1) -> Sum2/7
  8/1(Out1) -> Sum2/8
  21/1(Out1) -> Sum2/21
  20/1(Out1) -> Sum2/20
  18/1(Out1) -> Sum2/18
  17/1(Out1) -> Sum2/17
  16/1(Out1) -> Sum2/16
  15/1(Out1) -> Sum2/15
  14/1(Out1) -> Sum2/14
  13/1(Out1) -> Sum2/13
  12/1(Out1) -> Sum2/12
  11/1(Out1) -> Sum2/11
  10/1(Out1) -> Sum2/10
  9/1(Out1) -> Sum2/9
  In/1 -> Klasifikacia1/1
  Klasifikacia1/1 -> 1/Action
  Klasifikacia1/2 -> 2/Action
  Klasifikacia1/3 -> 3/Action
  Klasifikacia1/4 -> 4/Action
  Klasifikacia1/5 -> 5/Action
  Klasifikacia1/6 -> 6/Action
  Klasifikacia1/7 -> 7/Action
  Klasifikacia1/8 -> 8/Action
  Klasifikacia1/9 -> 9/Action
  Klasifikacia1/10 -> 10/Action
  Klasifikacia1/11 -> 11/Action
  Klasifikacia1/12 -> 12/Action
  Klasifikacia1/13 -> 13/Action
  Klasifikacia1/14 -> 14/Action
  Klasifikacia1/15 -> 15/Action
  Klasifikacia1/16 -> 16/Action
  Klasifikacia1/17 -> 17/Action
  Klasifikacia1/18 -> 18/Action
  Klasifikacia1/19 -> 19/Action
  Klasifikacia1/20 -> 20/Action
  Klasifikacia1/21 -> 21/Action
  Sum2/1 -> Out/1
  Klasifikacia1/22 -> Terminator1/1
  19/1(Out1) -> Sum2/19

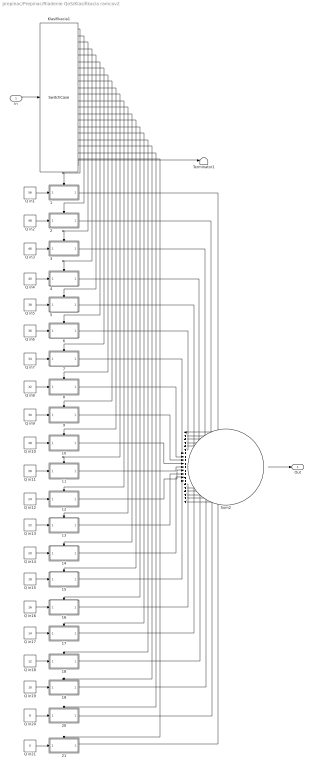
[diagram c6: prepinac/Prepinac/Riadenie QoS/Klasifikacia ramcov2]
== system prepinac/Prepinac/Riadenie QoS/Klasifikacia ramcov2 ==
  In : Inport  OutDataType=sfix(16)  OutScaling=2^0
  1 : Subsystem  TreatAsAtomicUnit=on
  10 : Subsystem  TreatAsAtomicUnit=on
  11 : Subsystem  TreatAsAtomicUnit=on
  12 : Subsystem  TreatAsAtomicUnit=on
  13 : Subsystem  TreatAsAtomicUnit=on
  14 : Subsystem  TreatAsAtomicUnit=on
  15 : Subsystem  TreatAsAtomicUnit=on
  16 : Subsystem  TreatAsAtomicUnit=on
  17 : Subsystem  TreatAsAtomicUnit=on
  18 : Subsystem  TreatAsAtomicUnit=on
  19 : Subsystem  TreatAsAtomicUnit=on
  2 : Subsystem  TreatAsAtomicUnit=on
  20 : Subsystem  TreatAsAtomicUnit=on
  21 : Subsystem  TreatAsAtomicUnit=on
  3 : Subsystem  TreatAsAtomicUnit=on
  4 : Subsystem  TreatAsAtomicUnit=on
  5 : Subsystem  TreatAsAtomicUnit=on
  6 : Subsystem  TreatAsAtomicUnit=on
  7 : Subsystem  TreatAsAtomicUnit=on
  8 : Subsystem  TreatAsAtomicUnit=on
  9 : Subsystem  TreatAsAtomicUnit=on
  Klasifikacia1 : SwitchCase  CaseConditions={0,8,10,12,14,16,18,20,22,24,26,28,30,32,34,36,38,40,46,48,56}
  Q in1 : Constant  Value=56  VectorParams1D=off  OutDataTypeMode=double  OutDataType=sfix(16)  OutScaling=2^0  OutDataTypeStr=double  SampleTime=-1
  Q in10 : Constant  Value=28  VectorParams1D=off  OutDataTypeMode=double  OutDataType=sfix(16)  OutScaling=2^0  OutDataTypeStr=double  SampleTime=-1
  Q in11 : Constant  Value=26  VectorParams1D=off  OutDataTypeMode=double  OutDataType=sfix(16)  OutScaling=2^0  OutDataTypeStr=double  SampleTime=-1
  Q in12 : Constant  Value=24  VectorParams1D=off  OutDataTypeMode=double  OutDataType=sfix(16)  OutScaling=2^0  OutDataTypeStr=double  SampleTime=-1
  Q in13 : Constant  Value=22  VectorParams1D=off  OutDataTypeMode=double  OutDataType=sfix(16)  OutScaling=2^0  OutDataTypeStr=double  SampleTime=-1
  Q in14 : Constant  Value=20  VectorParams1D=off  OutDataTypeMode=double  OutDataType=sfix(16)  OutScaling=2^0  OutDataTypeStr=double  SampleTime=-1
  Q in15 : Constant  Value=18  VectorParams1D=off  OutDataTypeMode=double  OutDataType=sfix(16)  OutScaling=2^0  OutDataTypeStr=double  SampleTime=-1
  Q in16 : Constant  Value=16  VectorParams1D=off  OutDataTypeMode=double  OutDataType=sfix(16)  OutScaling=2^0  OutDataTypeStr=double  SampleTime=-1
  Q in17 : Constant  Value=14  VectorParams1D=off  OutDataTypeMode=double  OutDataType=sfix(16)  OutScaling=2^0  OutDataTypeStr=double  SampleTime=-1
  Q in18 : Constant  Value=12  VectorParams1D=off  OutDataTypeMode=double  OutDataType=sfix(16)  OutScaling=2^0  OutDataTypeStr=double  SampleTime=-1
  Q in19 : Constant  Value=10  VectorParams1D=off  OutDataTypeMode=double  OutDataType=sfix(16)  OutScaling=2^0  OutDataTypeStr=double  SampleTime=-1
  Q in2 : Constant  Value=48  VectorParams1D=off  OutDataTypeMode=double  OutDataType=sfix(16)  OutScaling=2^0  OutDataTypeStr=double  SampleTime=-1
  Q in20 : Constant  Value=8  VectorParams1D=off  OutDataTypeMode=double  OutDataType=sfix(16)  OutScaling=2^0  OutDataTypeStr=double  SampleTime=-1
  Q in21 : Constant  Value=0  VectorParams1D=off  OutDataTypeMode=double  OutDataType=sfix(16)  OutScaling=2^0  OutDataTypeStr=double  SampleTime=-1
  Q in3 : Constant  Value=46  VectorParams1D=off  OutDataTypeMode=double  OutDataType=sfix(16)  OutScaling=2^0  OutDataTypeStr=double  SampleTime=-1
  Q in4 : Constant  Value=40  VectorParams1D=off  OutDataTypeMode=double  OutDataType=sfix(16)  OutScaling=2^0  OutDataTypeStr=double  SampleTime=-1
  Q in5 : Constant  Value=38  VectorParams1D=off  OutDataTypeMode=double  OutDataType=sfix(16)  OutScaling=2^0  OutDataTypeStr=double  SampleTime=-1
  Q in6 : Constant  Value=36  VectorParams1D=off  OutDataTypeMode=double  OutDataType=sfix(16)  OutScaling=2^0  OutDataTypeStr=double  SampleTime=-1
  Q in7 : Constant  Value=34  VectorParams1D=off  OutDataTypeMode=double  OutDataType=sfix(16)  OutScaling=2^0  OutDataTypeStr=double  SampleTime=-1
  Q in8 : Constant  Value=32  VectorParams1D=off  OutDataTypeMode=double  OutDataType=sfix(16)  OutScaling=2^0  OutDataTypeStr=double  SampleTime=-1
  Q in9 : Constant  Value=30  VectorParams1D=off  OutDataTypeMode=double  OutDataType=sfix(16)  OutScaling=2^0  OutDataTypeStr=double  SampleTime=-1
  Sum2 : Sum  Inputs=|+++++++++++++++++++++  OutDataType=sfix(16)  OutScaling=2^0
  Terminator1 : Terminator
  Out : Outport  OutDataType=sfix(16)  OutScaling=2^0
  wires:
  19/1(Out1) -> Sum2/19
  Klasifikacia1/22 -> Terminator1/1
  Sum2/1 -> Out/1
  Klasifikacia1/21 -> 21/Action
  Klasifikacia1/20 -> 20/Action
  Klasifikacia1/19 -> 19/Action
  Klasifikacia1/18 -> 18/Action
  Klasifikacia1/17 -> 17/Action
  Klasifikacia1/16 -> 16/Action
  Klasifikacia1/15 -> 15/Action
  Klasifikacia1/14 -> 14/Action
  Klasifikacia1/13 -> 13/Action
  Klasifikacia1/12 -> 12/Action
  Klasifikacia1/11 -> 11/Action
  Klasifikacia1/10 -> 10/Action
  Klasifikacia1/9 -> 9/Action
  Klasifikacia1/8 -> 8/Action
  Klasifikacia1/7 -> 7/Action
  Klasifikacia1/6 -> 6/Action
  Klasifikacia1/5 -> 5/Action
  Klasifikacia1/4 -> 4/Action
  Klasifikacia1/3 -> 3/Action
  Klasifikacia1/2 -> 2/Action
  Klasifikacia1/1 -> 1/Action
  In/1 -> Klasifikacia1/1
  9/1(Out1) -> Sum2/9
  10/1(Out1) -> Sum2/10
  11/1(Out1) -> Sum2/11
  12/1(Out1) -> Sum2/12
  13/1(Out1) -> Sum2/13
  14/1(Out1) -> Sum2/14
  15/1(Out1) -> Sum2/15
  16/1(Out1) -> Sum2/16
  17/1(Out1) -> Sum2/17
  18/1(Out1) -> Sum2/18
  20/1(Out1) -> Sum2/20
  21/1(Out1) -> Sum2/21
  8/1(Out1) -> Sum2/8
  7/1(Out1) -> Sum2/7
  6/1(Out1) -> Sum2/6
  5/1(Out1) -> Sum2/5
  Q in21/1 -> 21/1(In1)
  Q in20/1 -> 20/1(In1)
  Q in19/1 -> 19/1(In1)
  Q in18/1 -> 18/1(In1)
  Q in17/1 -> 17/1(In1)
  Q in16/1 -> 16/1(In1)
  Q in15/1 -> 15/1(In1)
  Q in14/1 -> 14/1(In1)
  Q in13/1 -> 13/1(In1)
  Q in12/1 -> 12/1(In1)
  Q in11/1 -> 11/1(In1)
  Q in10/1 -> 10/1(In1)
  Q in9/1 -> 9/1(In1)
  Q in8/1 -> 8/1(In1)
  Q in7/1 -> 7/1(In1)
  Q in6/1 -> 6/1(In1)
  Q in5/1 -> 5/1(In1)
  Q in4/1 -> 4/1(In1)
  Q in3/1 -> 3/1(In1)
  Q in2/1 -> 2/1(In1)
  Q in1/1 -> 1/1(In1)
  4/1(Out1) -> Sum2/4
  3/1(Out1) -> Sum2/3
  2/1(Out1) -> Sum2/2
  1/1(Out1) -> Sum2/1

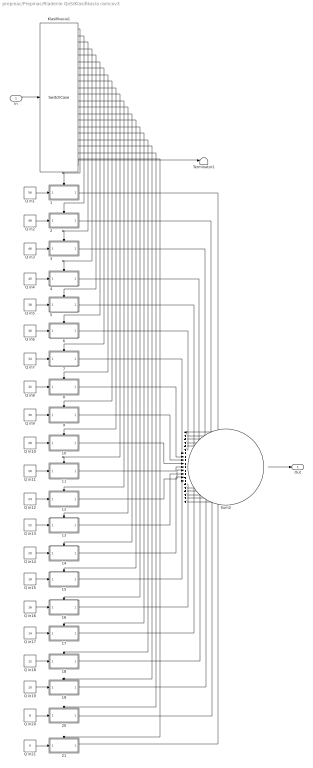
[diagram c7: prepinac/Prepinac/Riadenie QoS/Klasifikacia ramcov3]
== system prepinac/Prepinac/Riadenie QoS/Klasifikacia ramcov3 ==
  In : Inport  OutDataType=sfix(16)  OutScaling=2^0
  1 : Subsystem  TreatAsAtomicUnit=on
  10 : Subsystem  TreatAsAtomicUnit=on
  11 : Subsystem  TreatAsAtomicUnit=on
  12 : Subsystem  TreatAsAtomicUnit=on
  13 : Subsystem  TreatAsAtomicUnit=on
  14 : Subsystem  TreatAsAtomicUnit=on
  15 : Subsystem  TreatAsAtomicUnit=on
  16 : Subsystem  TreatAsAtomicUnit=on
  17 : Subsystem  TreatAsAtomicUnit=on
  18 : Subsystem  TreatAsAtomicUnit=on
  19 : Subsystem  TreatAsAtomicUnit=on
  2 : Subsystem  TreatAsAtomicUnit=on
  20 : Subsystem  TreatAsAtomicUnit=on
  21 : Subsystem  TreatAsAtomicUnit=on
  3 : Subsystem  TreatAsAtomicUnit=on
  4 : Subsystem  TreatAsAtomicUnit=on
  5 : Subsystem  TreatAsAtomicUnit=on
  6 : Subsystem  TreatAsAtomicUnit=on
  7 : Subsystem  TreatAsAtomicUnit=on
  8 : Subsystem  TreatAsAtomicUnit=on
  9 : Subsystem  TreatAsAtomicUnit=on
  Klasifikacia1 : SwitchCase  CaseConditions={0,8,10,12,14,16,18,20,22,24,26,28,30,32,34,36,38,40,46,48,56}
  Q in1 : Constant  Value=56  VectorParams1D=off  OutDataTypeMode=double  OutDataType=sfix(16)  OutScaling=2^0  OutDataTypeStr=double  SampleTime=-1
  Q in10 : Constant  Value=28  VectorParams1D=off  OutDataTypeMode=double  OutDataType=sfix(16)  OutScaling=2^0  OutDataTypeStr=double  SampleTime=-1
  Q in11 : Constant  Value=26  VectorParams1D=off  OutDataTypeMode=double  OutDataType=sfix(16)  OutScaling=2^0  OutDataTypeStr=double  SampleTime=-1
  Q in12 : Constant  Value=24  VectorParams1D=off  OutDataTypeMode=double  OutDataType=sfix(16)  OutScaling=2^0  OutDataTypeStr=double  SampleTime=-1
  Q in13 : Constant  Value=22  VectorParams1D=off  OutDataTypeMode=double  OutDataType=sfix(16)  OutScaling=2^0  OutDataTypeStr=double  SampleTime=-1
  Q in14 : Constant  Value=20  VectorParams1D=off  OutDataTypeMode=double  OutDataType=sfix(16)  OutScaling=2^0  OutDataTypeStr=double  SampleTime=-1
  Q in15 : Constant  Value=18  VectorParams1D=off  OutDataTypeMode=double  OutDataType=sfix(16)  OutScaling=2^0  OutDataTypeStr=double  SampleTime=-1
  Q in16 : Constant  Value=16  VectorParams1D=off  OutDataTypeMode=double  OutDataType=sfix(16)  OutScaling=2^0  OutDataTypeStr=double  SampleTime=-1
  Q in17 : Constant  Value=14  VectorParams1D=off  OutDataTypeMode=double  OutDataType=sfix(16)  OutScaling=2^0  OutDataTypeStr=double  SampleTime=-1
  Q in18 : Constant  Value=12  VectorParams1D=off  OutDataTypeMode=double  OutDataType=sfix(16)  OutScaling=2^0  OutDataTypeStr=double  SampleTime=-1
  Q in19 : Constant  Value=10  VectorParams1D=off  OutDataTypeMode=double  OutDataType=sfix(16)  OutScaling=2^0  OutDataTypeStr=double  SampleTime=-1
  Q in2 : Constant  Value=48  VectorParams1D=off  OutDataTypeMode=double  OutDataType=sfix(16)  OutScaling=2^0  OutDataTypeStr=double  SampleTime=-1
  Q in20 : Constant  Value=8  VectorParams1D=off  OutDataTypeMode=double  OutDataType=sfix(16)  OutScaling=2^0  OutDataTypeStr=double  SampleTime=-1
  Q in21 : Constant  Value=0  VectorParams1D=off  OutDataTypeMode=double  OutDataType=sfix(16)  OutScaling=2^0  OutDataTypeStr=double  SampleTime=-1
  Q in3 : Constant  Value=46  VectorParams1D=off  OutDataTypeMode=double  OutDataType=sfix(16)  OutScaling=2^0  OutDataTypeStr=double  SampleTime=-1
  Q in4 : Constant  Value=40  VectorParams1D=off  OutDataTypeMode=double  OutDataType=sfix(16)  OutScaling=2^0  OutDataTypeStr=double  SampleTime=-1
  Q in5 : Constant  Value=38  VectorParams1D=off  OutDataTypeMode=double  OutDataType=sfix(16)  OutScaling=2^0  OutDataTypeStr=double  SampleTime=-1
  Q in6 : Constant  Value=36  VectorParams1D=off  OutDataTypeMode=double  OutDataType=sfix(16)  OutScaling=2^0  OutDataTypeStr=double  SampleTime=-1
  Q in7 : Constant  Value=34  VectorParams1D=off  OutDataTypeMode=double  OutDataType=sfix(16)  OutScaling=2^0  OutDataTypeStr=double  SampleTime=-1
  Q in8 : Constant  Value=32  VectorParams1D=off  OutDataTypeMode=double  OutDataType=sfix(16)  OutScaling=2^0  OutDataTypeStr=double  SampleTime=-1
  Q in9 : Constant  Value=30  VectorParams1D=off  OutDataTypeMode=double  OutDataType=sfix(16)  OutScaling=2^0  OutDataTypeStr=double  SampleTime=-1
  Sum2 : Sum  Inputs=|+++++++++++++++++++++  OutDataType=sfix(16)  OutScaling=2^0
  Terminator1 : Terminator
  Out : Outport  OutDataType=sfix(16)  OutScaling=2^0
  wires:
  1/1(Out1) -> Sum2/1
  2/1(Out1) -> Sum2/2
  3/1(Out1) -> Sum2/3
  4/1(Out1) -> Sum2/4
  Q in1/1 -> 1/1(In1)
  Q in2/1 -> 2/1(In1)
  Q in3/1 -> 3/1(In1)
  Q in4/1 -> 4/1(In1)
  Q in5/1 -> 5/1(In1)
  Q in6/1 -> 6/1(In1)
  Q in7/1 -> 7/1(In1)
  Q in8/1 -> 8/1(In1)
  Q in9/1 -> 9/1(In1)
  Q in10/1 -> 10/1(In1)
  Q in11/1 -> 11/1(In1)
  Q in12/1 -> 12/1(In1)
  Q in13/1 -> 13/1(In1)
  Q in14/1 -> 14/1(In1)
  Q in15/1 -> 15/1(In1)
  Q in16/1 -> 16/1(In1)
  Q in17/1 -> 17/1(In1)
  Q in18/1 -> 18/1(In1)
  Q in19/1 -> 19/1(In1)
  Q in20/1 -> 20/1(In1)
  Q in21/1 -> 21/1(In1)
  5/1(Out1) -> Sum2/5
  6/1(Out1) -> Sum2/6
  7/1(Out1) -> Sum2/7
  8/1(Out1) -> Sum2/8
  21/1(Out1) -> Sum2/21
  20/1(Out1) -> Sum2/20
  18/1(Out1) -> Sum2/18
  17/1(Out1) -> Sum2/17
  16/1(Out1) -> Sum2/16
  15/1(Out1) -> Sum2/15
  14/1(Out1) -> Sum2/14
  13/1(Out1) -> Sum2/13
  12/1(Out1) -> Sum2/12
  11/1(Out1) -> Sum2/11
  10/1(Out1) -> Sum2/10
  9/1(Out1) -> Sum2/9
  In/1 -> Klasifikacia1/1
  Klasifikacia1/1 -> 1/Action
  Klasifikacia1/2 -> 2/Action
  Klasifikacia1/3 -> 3/Action
  Klasifikacia1/4 -> 4/Action
  Klasifikacia1/5 -> 5/Action
  Klasifikacia1/6 -> 6/Action
  Klasifikacia1/7 -> 7/Action
  Klasifikacia1/8 -> 8/Action
  Klasifikacia1/9 -> 9/Action
  Klasifikacia1/10 -> 10/Action
  Klasifikacia1/11 -> 11/Action
  Klasifikacia1/12 -> 12/Action
  Klasifikacia1/13 -> 13/Action
  Klasifikacia1/14 -> 14/Action
  Klasifikacia1/15 -> 15/Action
  Klasifikacia1/16 -> 16/Action
  Klasifikacia1/17 -> 17/Action
  Klasifikacia1/18 -> 18/Action
  Klasifikacia1/19 -> 19/Action
  Klasifikacia1/20 -> 20/Action
  Klasifikacia1/21 -> 21/Action
  Sum2/1 -> Out/1
  Klasifikacia1/22 -> Terminator1/1
  19/1(Out1) -> Sum2/19
